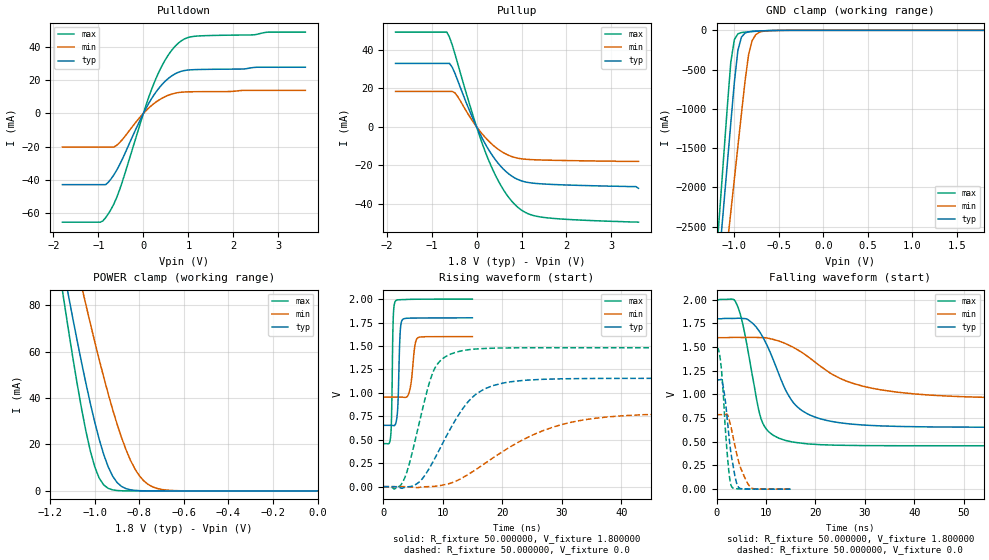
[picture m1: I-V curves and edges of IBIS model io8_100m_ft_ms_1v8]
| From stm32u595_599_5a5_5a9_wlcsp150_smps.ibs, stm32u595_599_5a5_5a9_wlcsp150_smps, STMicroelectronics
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|   Model io8_100m_ft_ms_1v8
[Model]  io8_100m_ft_ms_1v8
Model_type I/O
Polarity   Non-Inverting
Enable   Active-Low
Vinl =   0.540000V
Vinh =   1.260000V
Vmeas =  0.900000V
Cref =   50.000000pF
Rref =   100.000000M
Vref =   0.0V
C_comp   3.148300pF   3.147400pF   3.196500pF
[Temperature Range]   25.000000   0.140000k   -40.000000
[Pullup Reference]   1.800000V   1.600000V   2.000000V
[Pulldown Reference]   0.0V   0.0V   0.0V
[POWER Clamp Reference]   1.800000V   1.600000V   2.000000V
[GND Clamp Reference]   0.0V   0.0V   0.0V
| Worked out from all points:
|   slope of the pulldown table from 0 to 0.27 V, typ, clamps not added: 21.7 ohm
|   slope of the pullup table from 0 to 0.27 V, typ, clamps not added: 22.6 ohm
|   GND clamp passes 1 mA (typ) near -0.51 V on its own axis
|   POWER clamp passes 1 mA (typ) near -0.86 V on its own axis
|   rising waveform, R_fixture 50.000000, V_fixture 1.800000: 20-80 % time 319ps typ, 624ps min, 231ps max; typ from 0.654 V to 1.8 V
|   rising waveform, R_fixture 50.000000, V_fixture 0.0: 20-80 % time 6.48ns typ, 13.4ns min, 3.56ns max; typ from 0 V to 1.16 V
|   falling waveform, R_fixture 50.000000, V_fixture 1.800000: 20-80 % time 6.35ns typ, 13.5ns min, 3.35ns max; typ from 1.8 V to 0.654 V
|   falling waveform, R_fixture 50.000000, V_fixture 0.0: 20-80 % time 1.6ns typ, 2.38ns min, 1.18ns max; typ from 1.16 V to 0 V
[Pulldown]
|Voltage   I(typ)   I(min)   I(max)
-1.8V     -42.74mA   -20.21mA   -65.25mA
-960mV    -42.74mA   -20.21mA   -65.25mA
-780mV    -41.3mA    -20.21mA   -60.25mA
-660mV    -37mA      -20.2mA    -54.5mA
-540mV    -31.39mA   -17.82mA   -46.65mA
0V        0A         0A         10fA
240mV     11.28mA    6.002mA    18.38mA
480mV     19.18mA    10.02mA    31.83mA
780mV     24.67mA    12.5mA     42.21mA
960mV     25.9mA     12.9mA     45.21mA
1.2V      26.29mA    13.01mA    46.37mA
3.6V      27.67mA    13.81mA    48.75mA
[Pullup]
|Voltage   I(typ)   I(min)   I(max)
-1.8V     32.87mA    18.3mA     49.13mA
-660mV    32.87mA    18.3mA     49.13mA
-600mV    32.87mA    18.3mA     46.41mA
-480mV    27.73mA    17.56mA    37.8mA
-60mV     3.108mA    1.975mA    4.436mA
240mV     -10.82mA   -6.752mA   -15.73mA
420mV     -17.18mA   -10.64mA   -25.23mA
600mV     -22.1mA    -13.54mA   -32.82mA
960mV     -27.82mA   -16.55mA   -42.66mA
1.2V      -29.16mA   -17.09mA   -45.68mA
1.56V     -29.85mA   -17.38mA   -47.3mA
3.6V      -32mA      -18mA      -49.6mA
[GND_clamp]
|Voltage   I(typ)   I(min)   I(max)
-1.8V     -9.707A    -9.942A    -9.774A
-1.2V     -3.309A    -4.006A    -2.864A
-1.16V    -2.777A    -3.584A    -2.239A
-1.12V    -2.246A    -3.162A    -1.614A
-1.04V    -1.186A    -2.319A    -408.6mA
-1V       -663.9mA   -1.898A    -117.8mA
-960mV    -254mA     -1.478A    -45.14mA
-920mV    -86.03mA   -1.06A     -28.58mA
-840mV    -19.12mA   -308.9mA   -18.74mA
-800mV    -13.39mA   -130.8mA   -15.31mA
-720mV    -7.948mA   -25.37mA   -9.381mA
1.8V      0A         14.97nA    0A
[POWER_clamp]
|Voltage   I(typ)   I(min)   I(max)
-1.8V     470.8mA    433.7mA    554.6mA
-1.14V    95.25mA    122.7mA    82.82mA
-1.12V    84.97mA    114mA      70.27mA
-1.06V    55.51mA    88.42mA    35.67mA
-1.04V    46.34mA    80.15mA    25.76mA
-1V       29.51mA    64.13mA    10.3mA
-940mV    10.39mA    41.86mA    1.109mA
-900mV    3.624mA    28.77mA    182.8uA
-840mV    490.7uA    13.24mA    11.35uA
-800mV    116.8uA    6.532mA    1.77uA
-740mV    13.2uA     1.723mA    109.3nA
0V        0A         18.72nA    0A
[Ramp]
| variable   typ   min   max
dV/dt_r  0.69306/6.46801n   0.47204/13.34462n   0.88872/3.55831n
dV/dt_f  0.68762/6.34002n   0.38667/13.46325n   0.92481/3.34516n
R_load = 50.000000
[Rising Waveform]
R_fixture= 50.000000
V_fixture= 1.800000
V_fixture_min= 1.600000
V_fixture_max= 2.000000
|time   V(typ)   V(min)   V(max)
0s        654mV      955.4mV    458.7mV
1.231ns   653.9mV    955.4mV    544.1mV
1.652ns   651.1mV    955.4mV    1.794V
2.012ns   663.9mV    955.4mV    1.977V
2.432ns   866.8mV    955.4mV    1.991V
2.853ns   1.675V     955.2mV    1.993V
3.213ns   1.781V     954.1mV    1.994V
4.414ns   1.797V     1.026V     1.997V
5.766ns   1.798V     1.587V     1.998V
14.95ns   1.8V       1.6V       2V
[Rising Waveform]
R_fixture= 50.000000
V_fixture= 0.0
V_fixture_min= 0.0
V_fixture_max= 0.0
|time   V(typ)   V(min)   V(max)
0s        3.632uV    3.097uV    2.536uV
3.203ns   -17.22mV   118.3uV    44.34mV
6.206ns   60.77mV    -5.394mV   727.9mV
8.809ns   321.5mV    4.866mV    1.281V
13.21ns   819.6mV    91.76mV    1.449V
15.62ns   988.6mV    185.7mV    1.468V
20.22ns   1.106V     380.8mV    1.478V
27.03ns   1.145V     601.6mV    1.481V
35.44ns   1.154V     727.8mV    1.481V
99.7ns    1.155V     786.8mV    1.481V
[Falling Waveform]
R_fixture= 50.000000
V_fixture= 1.800000
V_fixture_min= 1.600000
V_fixture_max= 2.000000
|time   V(typ)   V(min)   V(max)
0s        1.8V       1.6V       2V
4.004ns   1.805V     1.603V     1.963V
5.405ns   1.802V     1.602V     1.721V
9.009ns   1.638V     1.601V     743.5mV
13.81ns   1.064V     1.541V     516.8mV
16.42ns   866.1mV    1.471V     490.9mV
20.02ns   759.5mV    1.339V     473mV
26.43ns   692mV      1.139V     462.8mV
36.64ns   663.1mV    1.024V     459mV
99.7ns    654mV      955.4mV    458.7mV
[Falling Waveform]
R_fixture= 50.000000
V_fixture= 0.0
V_fixture_min= 0.0
V_fixture_max= 0.0
|time   V(typ)   V(min)   V(max)
0s        1.155V     786.8mV    1.481V
750.8ps   1.156V     786.8mV    1.378V
1.321ns   1.091V     786.7mV    1.044V
1.802ns   923.8mV    788.2mV    623.7mV
2.282ns   679.5mV    779.1mV    303.4mV
2.673ns   482.1mV    711.9mV    109.5mV
3.033ns   343.6mV    630.3mV    28.79mV
4.234ns   38.87mV    340.7mV    3.883mV
6.757ns   1.791mV    26.77mV    738.7uV
14.95ns   3.632uV    3.097uV    2.536uV
